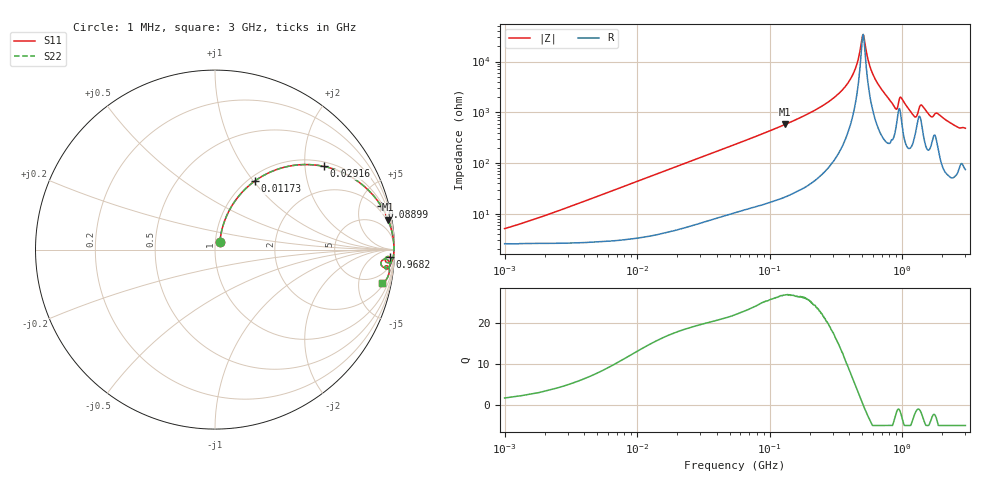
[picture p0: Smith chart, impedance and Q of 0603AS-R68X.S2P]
!s-Parameter Generated by FASTRON Sdn. Bhd.
!FASTRON P/N : 0603AS-R68X
!Keysight Technologies: E4991B_MY54100416_A.01.15
!Date created: Tue Oct 17 15:23:10 2023
!Version  : Rev01 Tue Oct 17 15:23:10 2023
!Data & Calibration Information:
!Freq	S11	S21	S12	S22
!PortZ  Port1:50+j0  Port2:50+j0
!When reading reference impedance value at option line is always used.
! Remarks : This data is being provided solely for informational purposes.
# Hz S dB R 50
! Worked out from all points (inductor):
!   1601 points, 1 MHz to 3 GHz, reference 50 ohm
!   read as one part in series: L = 700 nH near 1.796 MHz
!   highest Q = 26.9 at 130.8 MHz (marker M1), where L = 702 nH
!   self-resonance near 505.2 MHz
!   S11 on the Smith chart (normalised r, x): 1 MHz: 1.05, +0.09; 11.73 MHz: 1.07, +1.02; 29.16 MHz: 1.13, +2.50; 88.99 MHz: 1.30, +7.62; 968.2 MHz: 21, -34; 3 GHz: 2.49, -9.59
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1000000  -26.04 57.3  -0.23 -2.5  -0.23 -2.5  -26.04 57.3
3804036  -15.80 71.6  -0.34 -9.2  -0.34 -9.2  -15.80 71.6
1.172775e7  -7.08 59.8  -1.24 -26.2  -1.24 -26.2  -7.08 59.8
1.447069e7  -5.72 55.3  -1.68 -31.1  -1.68 -31.1  -5.72 55.3
2.915663e7  -2.36 37.5  -4.30 -49.6  -4.30 -49.6  -2.36 37.5
5.477226e7  -0.87 22.8  -8.22 -64.6  -8.22 -64.6  -0.87 22.8
8.899408e7  -0.37 14.5  -12.00 -73.2  -12.00 -73.2  -0.37 14.5
1.308271e8  -0.18 9.8  -15.41 -78.1  -15.41 -78.1  -0.18 9.8
2.083556e8  -0.07 5.6  -20.27 -82.1  -20.27 -82.1  -0.07 5.6
3.017325e8  -0.04 3.0  -25.55 -83.7  -25.55 -83.7  -0.04 3.0
3.855751e8  -0.03 1.6  -31.22 -82.5  -31.22 -82.5  -0.03 1.6
4.435663e8  -0.03 0.8  -37.27 -77.4  -37.27 -77.4  -0.03 0.8
5.077325e8  -0.03 -0.0  -50.71 0.5  -50.71 0.5  -0.03 -0.0
6.018993e8  -0.03 -1.0  -34.95 78.2  -34.95 78.2  -0.03 -1.0
7.925923e8  -0.07 -3.1  -25.38 79.3  -25.38 79.3  -0.07 -3.1
8.892696e8  -0.29 -4.3  -21.81 64.4  -21.81 64.4  -0.29 -4.3
9.682285e8  -0.23 -2.4  -26.18 56.8  -26.18 56.8  -0.23 -2.4
1.231095e9  -0.41 -6.1  -18.87 62.9  -18.87 62.9  -0.41 -6.1
1.402151e9  -0.28 -3.6  -23.11 61.4  -23.11 61.4  -0.28 -3.6
1.637435e9  -0.30 -6.4  -18.78 69.4  -18.78 69.4  -0.30 -6.4
1.837163e9  -0.26 -5.6  -19.88 70.0  -19.88 70.0  -0.26 -5.6
3e9  -0.44 -11.2  -14.15 70.0  -14.15 70.0  -0.44 -11.2
